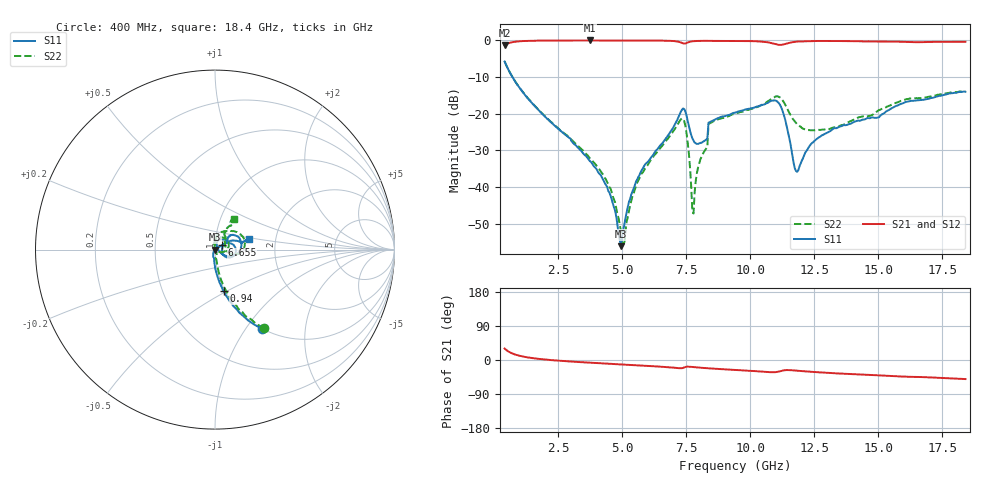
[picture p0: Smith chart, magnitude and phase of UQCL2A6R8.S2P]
! AVX Corporation
! Date:  10/27/06
! Part No:  UQCL2A6R8
! Description:  Ultra Low ESR Microwave capacitors
! Mounting Orientation:  Horizontal
# GHZ S DB R 50
! Freq  |S11|  S11 Ph  |S21|  S21 Ph  |S12|  S12 Ph  |S22|  S22 Ph
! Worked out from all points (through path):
!   401 points, 400 MHz to 18.4 GHz, reference 50 ohm
!   highest |S21| = -0.05 dB at 3.73 GHz (marker M1); lowest = -1.4 dB at 400 MHz (marker M2)
!   group delay of S21, straight-line fit = 8.92 ps
!   lowest |S11| = -56.1 dB at 4.945 GHz (marker M3), VSWR 1.00, Z = 50.1 - j0.11 ohm
!   |S11| at or under -10 dB: 703.7 MHz to end of sweep
!   |S22| runs from -55.8 to -5.8 dB; largest |S21 - S12| = 0.0052
!   S11 on the Smith chart (normalised r, x): 400 MHz: 1.00, -1.19; 940 MHz: 0.98, -0.48; 6.655 GHz: 1.08, +0.05; 18.4 GHz: 1.45, +0.18
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0.4  -5.80 -59.4  -1.41 30.3  -1.41 30.3  -5.75 -58.0
0.94  -12.53 -78.2  -0.30 11.9  -0.30 11.8  -12.53 -75.3
3.415  -30.30 -110.5  -0.05 -5.9  -0.05 -5.8  -29.71 -72.5
3.73  -32.91 -116.2  -0.05 -7.2  -0.05 -7.1  -32.10 -68.0
4.495  -41.52 -119.6  -0.06 -10.1  -0.06 -10.0  -40.00 -57.1
4.945  -56.09 -44.6  -0.06 -11.7  -0.06 -11.7  -51.92 -16.4
5.08  -50.14 4.8  -0.07 -12.2  -0.06 -12.2  -54.98 53.5
5.53  -38.56 29.8  -0.07 -13.8  -0.07 -13.8  -39.67 100.9
6.43  -29.11 32.2  -0.10 -17.3  -0.09 -17.3  -29.79 98.9
6.655  -27.08 33.3  -0.12 -18.3  -0.11 -18.2  -27.86 94.5
7.375  -18.57 -2.2  -0.86 -20.8  -0.83 -20.6  -21.43 26.5
7.51  -20.65 -29.3  -0.72 -17.8  -0.71 -17.7  -25.49 -13.1
7.69  -25.83 -30.8  -0.33 -18.2  -0.32 -18.1  -39.95 -26.6
7.78  -27.34 -21.9  -0.25 -18.8  -0.25 -18.7  -47.19 66.8
8.23  -27.29 17.3  -0.15 -21.3  -0.15 -21.2  -29.96 91.0
8.455  -22.13 36.9  -0.17 -22.5  -0.16 -22.4  -22.46 82.9
9.4  -19.73 42.8  -0.20 -25.9  -0.19 -25.8  -19.99 72.5
11.065  -16.79 3.8  -1.20 -31.1  -1.18 -31.0  -15.25 16.9
11.83  -35.84 27.7  -0.36 -28.2  -0.36 -28.1  -22.91 -10.5
12.415  -27.95 75.1  -0.20 -31.4  -0.20 -31.2  -24.51 9.7
15.43  -18.93 26.6  -0.34 -41.9  -0.32 -41.7  -17.84 60.7
18.4  -14.03 17.8  -0.40 -50.3  -0.40 -50.1  -13.93 57.6
